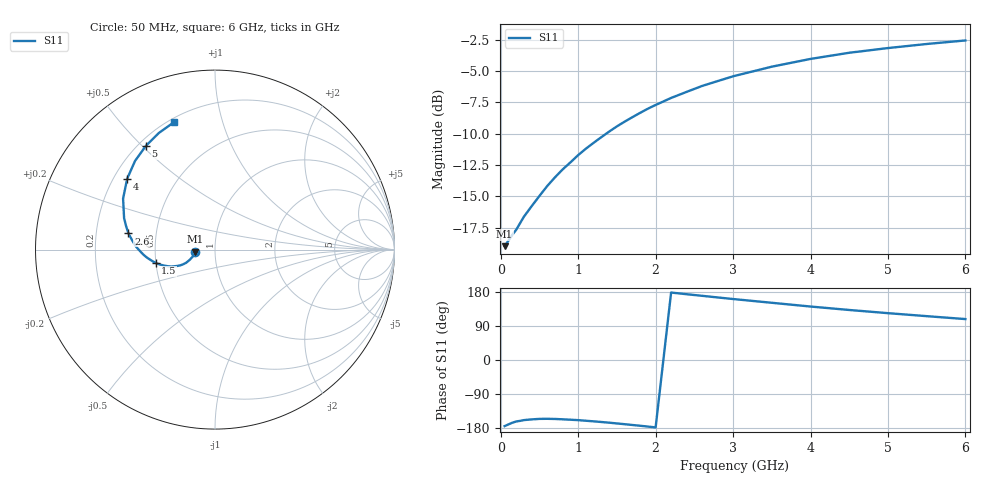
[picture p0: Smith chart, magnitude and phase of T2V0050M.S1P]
! SIEMENS Discrete & RF Semiconductors
! BAS70-04W
! Si Schottky Diode in SOT323
! IF = 50 mA
! S-Parameters:  November  1997
# GHz  S  MA  R  50
!  f  S11
! GHz  MAG  ANG
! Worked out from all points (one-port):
!   34 points, 50 MHz to 6 GHz, reference 50 ohm
!   lowest |S11| = -19.0 dB at 50 MHz (marker M1), VSWR 1.25, Z = 39.9 - j0.873 ohm
!   |S11| at or under -10 dB: start of sweep to 1.361 GHz
!   S11 on the Smith chart (normalised r, x): 50 MHz: 0.80, -0.02; 1.5 GHz: 0.50, -0.08; 2.6 GHz: 0.34, +0.08; 4 GHz: 0.25, +0.33; 5 GHz: 0.23, +0.51; 6 GHz: 0.22, +0.70
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0.05  0.1126 -174.5
0.15  0.125 -165.5
0.2  0.131 -162.2
0.3  0.1477 -158.6
0.4  0.1627 -156.7
0.5  0.1787 -155.4
0.6  0.1956 -155.2
0.7  0.2119 -155.6
0.8  0.228 -156.5
1  0.2599 -158.7
1.1  0.2757 -160.3
1.3  0.3067 -163.6
1.4  0.3226 -165.4
1.5  0.3383 -167.4
1.6  0.3535 -169.4
1.8  0.3832 -173.5
1.9  0.3981 -175.7
2.2  0.4394 178.0
2.4  0.4646 173.6
2.6  0.4905 169.4
2.8  0.5129 165.1
3  0.536 160.9
3.5  0.5855 151.0
4  0.6288 141.1
4.5  0.6654 132.0
5  0.6947 123.6
5.5  0.7212 115.7
6  0.745 108.0
